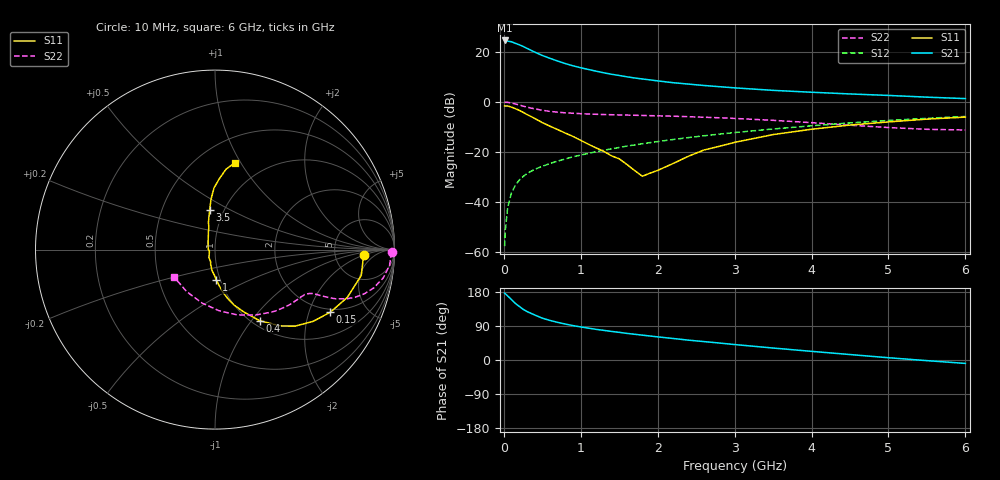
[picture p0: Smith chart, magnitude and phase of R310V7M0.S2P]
! SIEMENS Small Signal Semiconductors
! BFR181
! Si NPN RF Bipolar Junction Transistor in SOT23
! VCE = 10 V  IC = 7 mA
! Common Emitter S-Parameters:  May  1996
# GHz  S  MA  R  50
!  f  S11  S21  S12  S22
! GHz  MAG  ANG  MAG  ANG  MAG  ANG  MAG  ANG
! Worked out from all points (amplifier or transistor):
!   36 points, 10 MHz to 6 GHz, reference 50 ohm
!   highest |S21| = 24.6 dB at 10 MHz (marker M1)
!   |S21| within 3 dB of that: start of sweep to 289.7 MHz
!   unconditionally stable (mu >= 1): 1.063 GHz to 3.034 GHz
!   at 250 MHz: K = 0.49, MSG = 26.0 dB, |S12| = -29.9 dB
!   at 1.4 GHz: K = 1.04, MAG = 13.7 dB, |S12| = -18.8 dB
!   at 6 GHz: K = 0.87, MSG = 3.6 dB, |S12| = -5.8 dB
!   S11 on the Smith chart (normalised r, x): 10 MHz: 10, -2; 150 MHz: 1.86, -2.79; 400 MHz: 1.08, -1.10; 1 GHz: 0.96, -0.34; 3.5 GHz: 0.86, +0.40; 6 GHz: 0.74, +0.94
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0.01  0.8282 -2.1  16.91 176.6  0.0013 87.4  0.986 -0.9
0.02  0.827 -4.0  16.59 174.6  0.0028 77.8  0.9806 -2.0
0.05  0.8277 -10.0  16.39 169.1  0.0077 84.1  0.9769 -5.1
0.1  0.7836 -19.9  15.93 159.3  0.0153 79.1  0.9504 -9.6
0.15  0.7305 -28.6  14.84 149.4  0.0214 74.7  0.9093 -13.6
0.2  0.6771 -36.2  13.88 141.5  0.0272 72.3  0.8678 -16.5
0.25  0.6178 -43.6  12.86 133.9  0.032 69.0  0.8243 -18.8
0.3  0.5604 -49.4  11.76 128.0  0.0368 68.8  0.7853 -20.4
0.4  0.4674 -57.9  9.936 118.9  0.0447 66.9  0.7259 -22.2
0.5  0.3849 -65.0  8.473 110.4  0.0514 66.2  0.6793 -23.0
0.6  0.3265 -71.1  7.424 104.4  0.0586 66.3  0.6452 -23.5
0.7  0.2787 -75.7  6.552 99.3  0.0653 66.5  0.621 -23.8
0.8  0.2371 -80.0  5.822 94.8  0.0722 66.1  0.6035 -24.0
1  0.1702 -87.5  4.81 87.2  0.0863 66.5  0.5806 -24.9
1.1  0.1423 -91.4  4.444 84.1  0.0933 66.6  0.5716 -25.5
1.4  0.0832 -107.2  3.566 75.4  0.115 66.4  0.5535 -27.7
1.8  0.0325 -162.3  2.87 65.6  0.1454 65.0  0.5355 -31.6
2.2  0.0585 131.6  2.419 56.8  0.1767 63.0  0.5167 -36.5
3.5  0.2216 97.8  1.699 31.6  0.2869 53.1  0.4275 -58.6
4.5  0.3438 90.9  1.44 14.4  0.3793 42.8  0.3412 -86.3
5.5  0.4517 82.2  1.242 -1.7  0.469 30.8  0.2825 -123.9
6  0.4956 77.2  1.163 -9.0  0.5108 24.2  0.274 -145.5
